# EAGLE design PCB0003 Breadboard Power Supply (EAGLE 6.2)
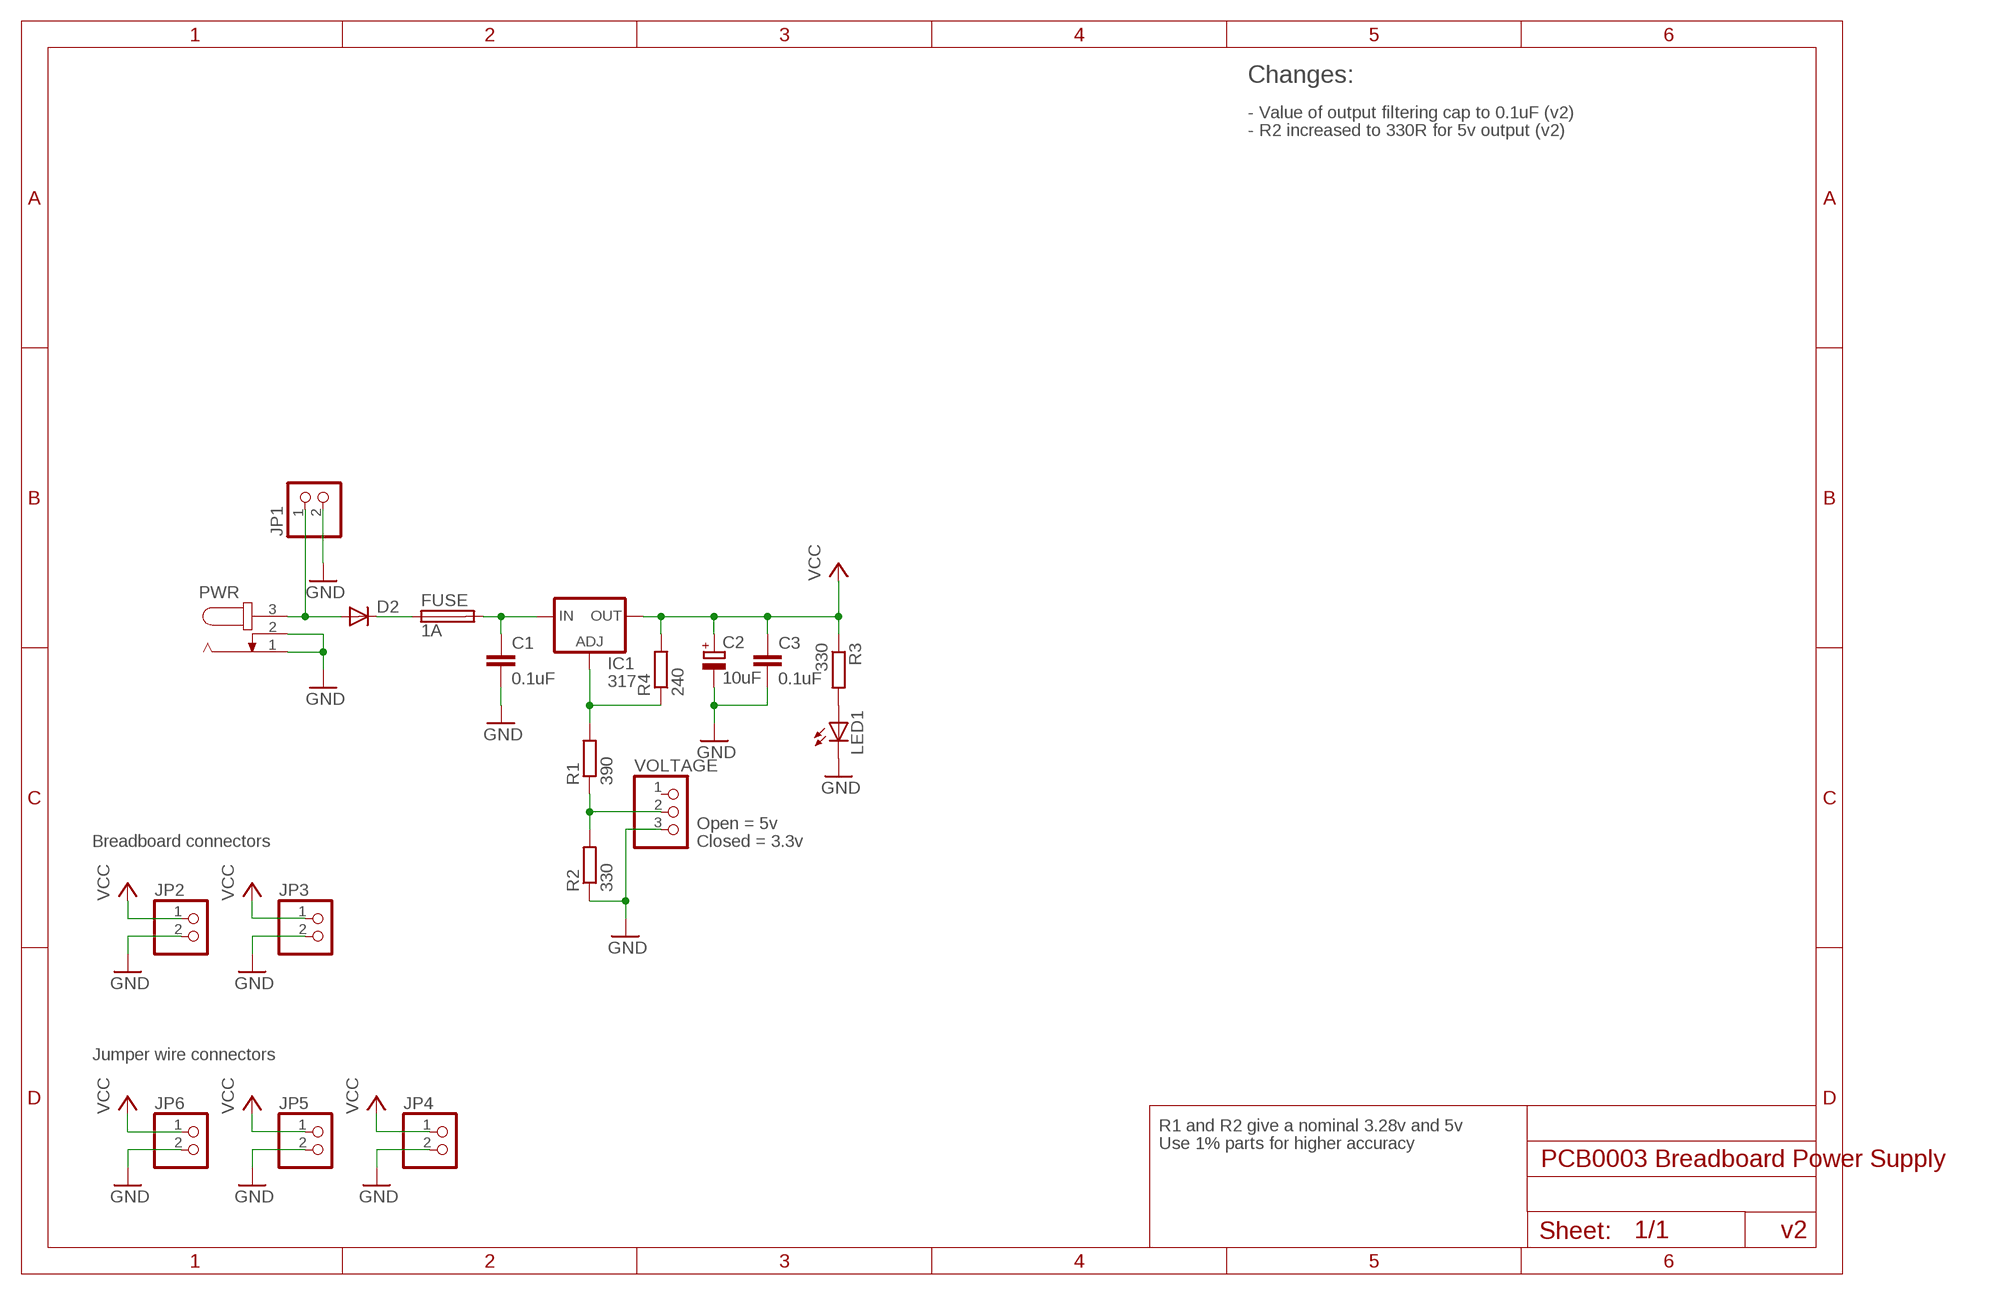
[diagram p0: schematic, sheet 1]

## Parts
C1  0.1uF  C-EU025_050-025X075  [C025_050-025X075]
C2  10uF  CPOL-EUE2-4  [E2-4]
C3  0.1uF  C-EU025_050-025X075  [C025_050-025X075]
D2  DIODE-C1702-05  [C1702-05]
FUSE  1A  TE5  [TE5]
IC1  317  LM317TS  [317TS]
JP1  PINHD1X2  [PINHD1X02]
JP2  PINHD-1X2  [1X02]
JP3  PINHD-1X2  [1X02]
JP4  PINHD-1X2  [1X02]
JP5  PINHD-1X2  [1X02]
JP6  PINHD-1X2  [1X02]
LED1  LED3MM  [LED3MM]
PWR  JACK-PLUG  [SPC4077-BIG-HOLES]
R1  390  R-EU_0207/10  [0207/10]
R2  330  R-EU_0207/10  [0207/10]
R3  330  R-EU_0207/10  [0207/10]
R4  240  R-EU_0207/10  [0207/10]
VOLTAGE  PINHD-1X3  [1X03]

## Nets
GND: C1.2 C2.- C3.2 JP1.2 JP2.2 JP3.2 JP4.2 JP5.2 JP6.2 LED1.K(C) PWR.1 PWR.2 R2.1 VOLTAGE.3
N$1: C1.1 FUSE.2 IC1.3(IN)
N$2: D2.C FUSE.1
N$3: IC1.1(ADJ) R1.2 R4.1
N$4: R1.1 R2.2 VOLTAGE.2
N$5: LED1.A R3.2
N$6: D2.A JP1.1 PWR.3
VCC: C2.+ C3.1 IC1.2(OUT) JP2.1 JP3.1 JP4.1 JP5.1 JP6.1 R3.1 R4.2
Unconnected: VOLTAGE.1

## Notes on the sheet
- Changes:
- - Value of output filtering cap to 0.1uF (v2)
- - R2 increased to 330R for 5v output (v2)
- Open = 5v
- Breadboard connectors | Closed = 3.3v
- Jumper wire connectors
- R1 and R2 give a nominal 3.28v and 5v
- Use 1% parts for higher accuracy
- v2

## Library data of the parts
C1 C3 = rcl:C-EU: CAPACITOR, European symbol
C2 = resistor:CPOL-EU: POLARIZED CAPACITOR, European symbol
D2 = diode:DIODE-: DIODE
FUSE = fuse:TE5: FUSE
IC1 = v-reg:LM317TS: VOLTAGE REGULATOR
JP1 = edeca:PINHD1X2
JP2-JP6 = pinhead:PINHD-1X2: PIN HEADER
LED1 = led:LED: LED
PWR = David's Eagle Library:JACK-PLUG: DC POWER JACK Power Jack, DC, Right Angle, Through Hole, Rated 5A at 16VDC, PC Terminals Distributor: Farnell (www.Farnell.de) Drawing: 84N1161.pdf / 84N1162.pdf Manufacturer: SPC Technology (www.spctechnology.com) Type: SPC4077 / SPC 4078
R1-R4 = resistor:R-EU_: RESISTOR, European symbol
VOLTAGE = pinhead:PINHD-1X3: PIN HEADER

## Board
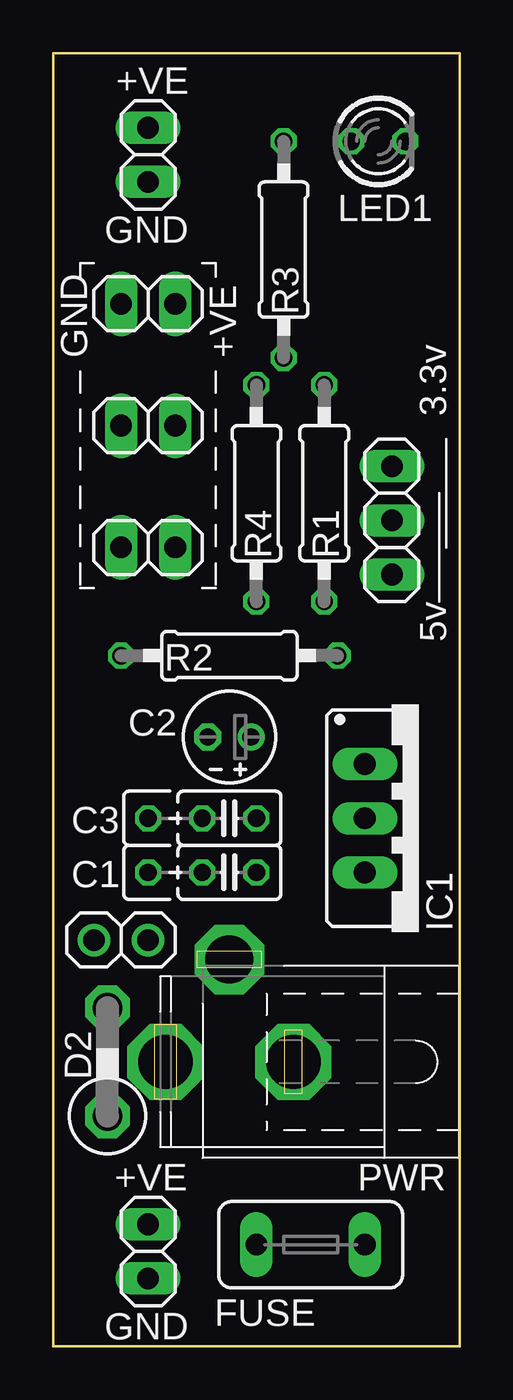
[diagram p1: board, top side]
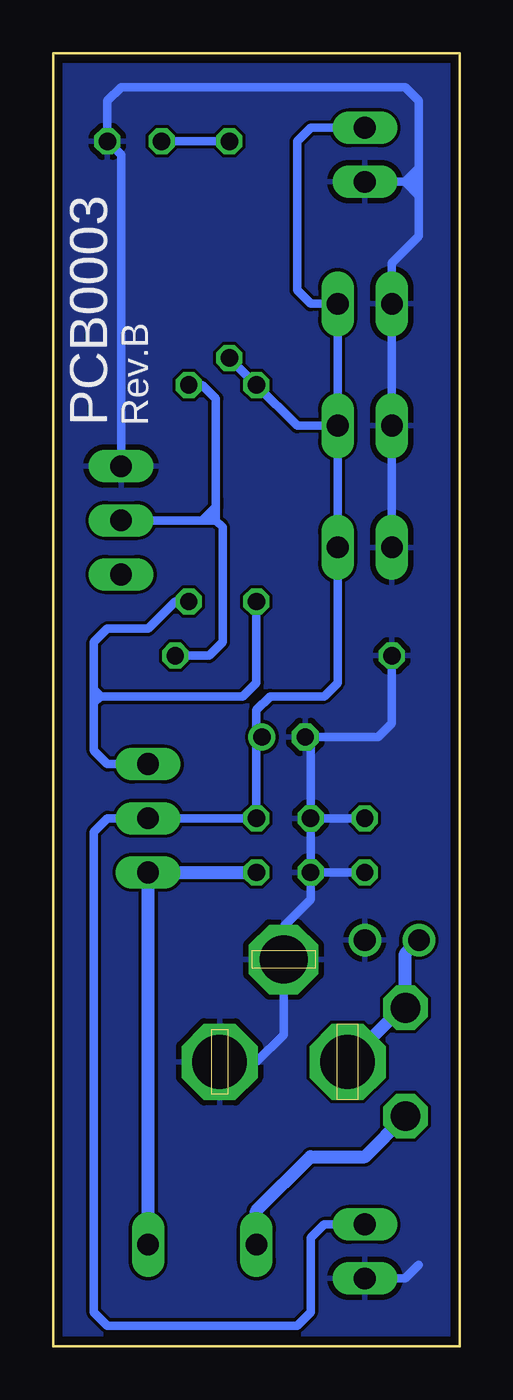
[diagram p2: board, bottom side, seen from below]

Size 19.05 x 60.64 mm. Coordinates in mm from the lower left corner, seen from the top.
Outline: 0,60.64 0,0 19.05,0 19.05,60.64 0,60.64
Copper layers (1*16): Top 0.0356mm / dielectric 1.5011mm / Bottom 0.0356mm
Design rules: minimum track width 6mil, minimum drill 13mil, track to track 6mil, track to pad 6mil, pad to pad 6mil, via to via 6mil, smd to smd 6mil, copper to edge 15mil, drill to drill 6mil, minimum pad ring 7mil, minimum via ring 7mil, stop-mask expansion 4mil, vias tented up to drill 0mil, thermal gap 10mil

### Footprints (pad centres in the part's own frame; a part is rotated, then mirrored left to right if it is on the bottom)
C025_050-025X075 = drill 0.813 octagon: 1 -1.27,0; 2 1.27,0; 3 3.81,0
E2-4 = drill 0.813 pad 1.27: + -1.016,0 | drill 0.813 pad 1.27 octagon: - 1.016,0
C1702-05 = drill 1.397 octagon: A 2.54,0; C -2.54,0
TE5 = drill 1.016 long: 1 -2.54,0; 2 2.54,0
317TS = drill 1.016 long: 1 -2.54,-2.54; 2 0,-2.54; 3 2.54,-2.54
PINHD1X02 = drill 1.016: 1 -1.27,0; 2 1.27,0
1X02 = drill 1.016 long: 1 -1.27,0; 2 1.27,0
LED3MM = drill 0.813 octagon: A -1.27,0; K 1.27,0
SPC4077-BIG-HOLES = drill 2.55 octagon: 1 -3,0; 3 3,0 | drill 2.25 octagon: 2 0,-4.8
0207/10 = drill 0.813 octagon: 1 -5.08,0; 2 5.08,0
1X03 = drill 1.016 long: 1 -2.54,0; 2 0,0; 3 2.54,0

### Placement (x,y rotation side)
C1  8.26,22.23 180 top
C2  8.26,28.57 180 top
C3  8.26,24.77 180 top
D2  2.54,13.34 90 top
FUSE  12.06,4.76 0 top
IC1  17.14,24.77 270 top
JP1  3.17,19.05 0 top
JP2  4.45,55.88 270 top
JP3  4.45,4.45 270 top
JP4  4.45,48.9 180 top
JP5  4.45,43.18 180 top
JP6  4.45,37.47 180 top
LED1  15.24,56.52 0 top
PWR  8.26,13.34 180 top
R1  12.7,40.01 270 top
R2  8.26,32.38 0 top
R3  10.79,51.44 90 top
R4  9.53,40.01 90 top
VOLTAGE  15.88,38.73 90 top

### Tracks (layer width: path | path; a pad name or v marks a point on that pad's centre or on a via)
GND
  Bottom 0.406: PWR.1 9.53,13.34 8.26,14.61 PWR.2 8.26,19.68 6.99,20.95 C1.2 | C1.2 C3.2 | C3.2 6.99,28.32 C2.- 3.81,28.57 3.17,29.21 R2.1 | C3.2 4.45,24.77 | C1.2 4.45,22.23 | JP3.2 2.54,3.17 1.91,3.81 | JP6.2 JP5.2 JP4.2 3.17,50.8 1.91,52.07 1.91,53.98 | 1.91,55.24 1.91,58.42 2.54,59.05 15.88,59.05 16.51,58.42 LED1.K 15.88,55.88 VOLTAGE.3 | 2.54,54.61 1.91,55.24 | 2.54,54.61 JP2.2 | 1.91,54.61 1.91,55.24 | 1.91,53.98 2.54,54.61 | 1.91,53.98 1.91,54.61 | 2.54,54.61 1.91,54.61
  pour Bottom: 0,60.64 19.05,60.64 19.05,0 0,0
N$1
  Bottom 0.61: FUSE.2 IC1.3 C1.1
N$2
  Bottom 0.61: FUSE.1 9.53,6.35 6.99,8.89 4.45,8.89 D2.C
N$3
  Bottom 0.406: IC1.1 16.51,27.3 17.14,27.94 17.14,30.16 | R4.1 9.53,31.11 10.16,30.48 16.83,30.48 | R1.2 13.34,34.92 14.61,33.66 16.51,33.66 17.14,33.02 17.14,30.8 | 17.14,30.16 17.14,30.48 | 17.14,30.48 16.83,30.48 | 16.83,30.48 17.14,30.8 | 17.14,30.48 17.14,30.8 | 17.14,30.16 16.83,30.48
N$4
  Bottom 0.406: R2.2 11.75,32.38 11.11,33.02 11.11,38.42 11.43,38.73 | R1.1 12.06,45.09 11.43,44.45 11.43,39.69 11.43,39.37 | 12.06,38.73 VOLTAGE.2 | 12.06,38.73 11.43,39.37 | 11.43,38.73 12.06,38.73 | 11.43,38.73 11.43,39.37
N$5
  Bottom 0.406: R3.2 LED1.A
N$6
  Bottom 0.61: PWR.3 2.71,15.88 D2.A 2.54,18.41 JP1.1
VCC
  Bottom 0.406: JP3.1 6.35,5.71 6.99,5.08 6.99,1.59 7.62,0.95 16.51,0.95 17.14,1.59 17.14,24.13 16.51,24.77 IC1.2 C3.1 9.53,28.57 | JP5.1 JP6.1 5.71,31.11 6.35,30.48 8.89,30.48 9.53,29.84 9.53,28.57 | JP5.1 JP4.1 6.99,48.9 7.62,49.53 7.62,56.52 6.99,57.15 JP2.1 | R3.1 R4.2 7.62,43.18 JP5.1 | 9.53,28.57 C2.+

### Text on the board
tPlace: +VE | GND | 3.3v | GND | +VE | 5v | +VE | GND
bNames: Rev.B | PCB0003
